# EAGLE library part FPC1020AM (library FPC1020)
FPC1020AM Fingerprint Sensor flexible cable Connector: Hirose Part Number: BM10NB(0.8)-16DS-0.4V(51)
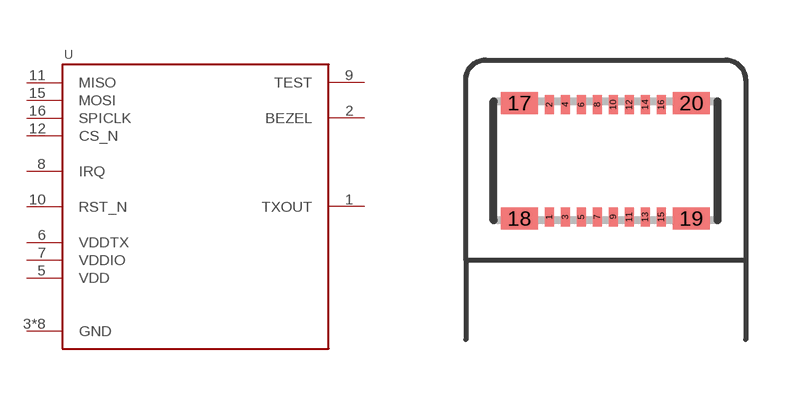
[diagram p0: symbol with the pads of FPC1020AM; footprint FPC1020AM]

Designator prefix -

## FPC1020AM  [FPC1020AM]
1  TXOUT  out
2  BEZEL
3  GND  pwr
4  GND  pwr
5  VDD  pwr
6  VDDTX  pwr
7  VDDIO  pwr
8  IRQ  out
9  TEST
10  RST_N  in
11  MISO
12  CS_N  in
13  GND  pwr
14  GND  pwr
15  MOSI
16  SPICLK  in
17  GND  pwr
18  GND  pwr
19  GND  pwr
20  GND  pwr

## Footprint FPC1020AM (pad centres in mm)
FCP1020AM Fingerprint Sensor flexible cable connector Connector Hirose Part Number BM10NB(0.8)-16DS-0.4V(51)
smd 0.23 x 0.47: 1 2.094,-3.929; 2 2.094,-1.119; 3 2.494,-3.929; 4 2.494,-1.119; 5 2.894,-3.929; 6 2.894,-1.119; 7 3.294,-3.929; 8 3.294,-1.119; 9 3.694,-3.929; 10 3.694,-1.119; 11 4.094,-3.929; 12 4.094,-1.119; 13 4.494,-3.929; 14 4.494,-1.119; 15 4.894,-3.929; 16 4.894,-1.119
smd 0.92 x 0.55: 17 1.344,-1.079; 18 1.344,-3.969; 19 5.644,-3.969; 20 5.644,-1.079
